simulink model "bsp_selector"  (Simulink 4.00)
settings: Solver=ode45  SolverMode=SingleTasking  StartTime=0.0  StopTime=10.0  FixedStep=0.01  RelTol=1e-3

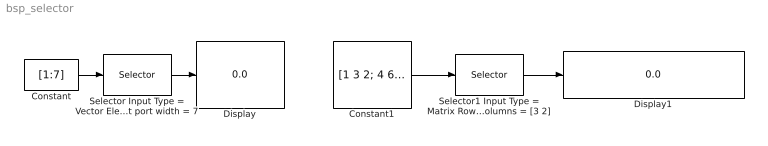
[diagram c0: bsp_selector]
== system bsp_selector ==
  Constant : Constant  Value=[1:7]
  Constant1 : Constant  Value=[1 3 2; 4 6 5; 8 10 9]  VectorParams1D=off
  Display : Display
  Display1 : Display
  Selector Input Type = Vector Elements = [1 3 6] Input port width = 7 : Selector  InputType=Vector  ElementSrc=Internal  Elements=[1 3 6]  RowSrc=Internal  Rows=1  ColumnSrc=Internal  Columns=1  InputPortWidth=7
  Selector1 Input Type = Matrix Rows = [2 3] Columns = [3 2] : Selector  InputType=Matrix  ElementSrc=Internal  Elements=[1 3 6]  RowSrc=Internal  Rows=[2 3]  ColumnSrc=Internal  Columns=[3 2]  InputPortWidth=7
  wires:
  Selector Input Type = Vector Elements = [1 3 6] Input port width = 7/1 -> Display/1
  Constant/1 -> Selector Input Type = Vector Elements = [1 3 6] Input port width = 7/1
  Constant1/1 -> Selector1 Input Type = Matrix Rows = [2 3] Columns = [3 2]/1
  Selector1 Input Type = Matrix Rows = [2 3] Columns = [3 2]/1 -> Display1/1
